(* This function block implements IEC60870-5-101 slave services *)
FUNCTION_BLOCK FB_IEC870_5_101SServices
VAR_IN_OUT
	stProcData 			: ST_IEC870_5_101SProcData;(* Process data send to or received from IEC 60870-5-101 slave device *)
	sysPara 			: ST_IEC870_5_101SSysPara;(* Local slave system parameters *)
	buffer				: ST_IEC870_5_101TBuffer;(* RX/TX buffer *)
	fbClock				: FB_LocalSystemTime;(* Internal clock: Local windows system time *)
	fbLog				: FB_IEC870_DebugLogFifo;(* Simple log buffer. We store/log here all our received slave data and other messages (for demonstration purpose only) *)
	bReset				: BOOL;(* Rising edge at this input resets service execution *)
END_VAR
VAR
	eState				: E_IEC870_5_101SState := e101SState_Init;(* Service/device execution state *)
	fbBuffer			: FB_IEC870_5_101TBufferCtrl; (* RX/TX buffer control function block *)
	txAsdu 				: ST_IEC870_5_101AOGen; (* Temp. asdu to send *)
	rxAsdu 				: ST_IEC870_5_101AOGen; (* Temp. received asdu *)
	fbSetLocalTime		: NT_SetLocalTime;

	fbCyclicTimer		: TON;(* Cyclic data timer *)
	fbCoroTimer			: TON;(* Local freeze/reset timer *)
	bGeninWait			: BOOL;(* TRUE => General interrogation in progress *)
	bCoroWait	 		: BOOL;(* TRUE => Counter interrogation in progress *)
	bEndOfInit			: BOOL;(* TRUE => End of initialization allready done *)

	st100 				: ST_IEC870_5_101SPendingState;(* Single point status flags *)
	st101 				: ST_IEC870_5_101SPendingState;(* Single point status flags *)
	st102 				: ST_IEC870_5_101SPendingState;(* Single point status flags *)
	st200 				: ST_IEC870_5_101SPendingState;(* Double point status flags *)
	st300 				: ST_IEC870_5_101SPendingState;(* Step position information status flags *)
	st400 				: ST_IEC870_5_101SPendingState;(* Bitstring status flags *)
	st500 				: ST_IEC870_5_101SPendingState;(* Measured value, normalized value status flags *)
	st600 				: ST_IEC870_5_101SPendingState;(* Measured value, scalled value status flags *)
	st700 				: ST_IEC870_5_101SPendingState;(* Measured value, short floating point number status flags *)
	st800 				: ST_IEC870_5_101SPendingState;(* Binary counter status flags *)
	st801 				: ST_IEC870_5_101SPendingState;(* Binary counter status flags *)
	st802 				: ST_IEC870_5_101SPendingState;(* Binary counter status flags *)
	
	stTxProcData		: ST_IEC870_5_101SProcData;
	
	(* Temporary variables *)
	tT56_new			: T_CP56Time2a;(* 56 bit time tag value *)
	tT56_old			: T_CP56Time2a;(* 56 bit time tag value *)
	tT24				: T_CP24Time2a;(* 24 bit time tag value *)
	tT56				: T_CP56Time2a;(* 56 bit time tag value *)
	stSiq				: ST_IEC870_5_101SIQ;(* Single point information + quality descriptor *)
	stDiq				: ST_IEC870_5_101DIQ;(* Double point information + quality descriptor *)
	stQds				: ST_IEC870_5_101QDS;(* Measured value quality descriptor *)
	stQcr				: ST_IEC870_5_101QCR;(* Binary counter quality descriptor *)

	nCoi				: BYTE;(* Cause of initialization *)
	eCoi				: E_IEC870_5_101COI := eIEC870_COI_LOCAL_POWER_ON;(* Cause of initialization as enumerated type *)
	
	nQoi				: BYTE;(* Qualifier of interrogation command *)	
	eQoi				: E_IEC870_5_101QOI;(* Qualifier of interrogation command as enumerated type *)
	
	nQcc				: BYTE;(* Qualifier of counter interrogation command *)
	eFrz				: E_IEC870_5_101FRZ;(* Counter interrogation freeze/reset qualifier *)
	eRqt				: E_IEC870_5_101RQT;(* Counter interrogation request qualifier *)

	nVti				: BYTE;(* Value with transient state indication *)
	nBsi				: DWORD;(* Bitstring information *)
	nNva				: WORD;(* Normalized value *)
	nSva				: INT;(* Scalled value *)
	fR32				: REAL;(* Short floating point value *)
	nBcr				: DINT;(* Binary counter reading *)
	
	nSco				: BYTE;(* Single command state + qualifier *)
	eScs				: E_IEC870_5_101SCS;(* Single command state *)
	
	nDco				: BYTE;(* Double command state + qualifier *)
	eDcs				: E_IEC870_5_101DCS;(* Double command state *)
	
	nRco				: BYTE;(* Regulating step command + qualifier *)
	eRcs				: E_IEC870_5_101RCS;(* Regulating step command *)
	
	eQu					: E_IEC870_5_101QU;(* Regulating step command qualifier *)
	nQos				: BYTE;(* Qualifier of setpoint command + select/execute flag *)
	eQl					: E_IEC870_5_101QL;(* Qualifier of setpoint command *)
	nFbp				: WORD := 16#55AA;(* Test command frame bit pattern activation data *)
	bSE					: BOOL;(* Select/execute flag (TRUE => Select, FALSE => Execute) *)
END_VAR

(* Please don't use the SIZEOF operator with CP56Time2a or CP24Time2a data type.
Because of the data alignment SIZEOF( tT56 ) or SIZEOF( tT24 ) leads to incorrect size. *)

IF bReset THEN(* Reset service execution *)
	bReset 	:= FALSE;
	MEMSET( ADR( st100 ), 0, SIZEOF( st100 ) );
	MEMSET( ADR( st101 ), 0, SIZEOF( st101 ) );
	MEMSET( ADR( st102 ), 0, SIZEOF( st102 ) );
	MEMSET( ADR( st200 ), 0, SIZEOF( st200 ) );
	MEMSET( ADR( st300 ), 0, SIZEOF( st300 ) );
	MEMSET( ADR( st400 ), 0, SIZEOF( st400 ) );
	MEMSET( ADR( st500 ), 0, SIZEOF( st500 ) );
	MEMSET( ADR( st600 ), 0, SIZEOF( st600 ) );
	MEMSET( ADR( st700 ), 0, SIZEOF( st700 ) );
	MEMSET( ADR( st800 ), 0, SIZEOF( st800 ) );
	MEMSET( ADR( st801 ), 0, SIZEOF( st801 ) );
	MEMSET( ADR( st802 ), 0, SIZEOF( st802 ) );
	fbCyclicTimer( IN := FALSE );(* Reset timer *)
	fbCoroTimer( IN := FALSE );(* Reset timer *)
	bGeninWait := FALSE;(* Reset flag *)
	bCoroWait := FALSE;(* Reset flag *)
	bEndOfInit := FALSE;(* Reset flag *)
	eState := e101SState_Init;
END_IF

(*-----------------------------------------------------------------------------------------*)
(* Simple implementation of cyclic data transfer *)
fbCyclicTimer( IN := sysPara.bCyclic, PT := sysPara.tCyclic );
IF fbCyclicTimer.Q THEN
	fbCyclicTimer( IN := FALSE ); 
	fbCyclicTimer( IN := sysPara.bCyclic );
	(* Set flags to force monitoring data to send cyclic data *)
	st100.bCyclic := TRUE;
	st101.bCyclic := TRUE;
	st102.bCyclic := TRUE;
	st200.bCyclic := TRUE;
	st300.bCyclic := TRUE;
	st400.bCyclic := TRUE;
	st500.bCyclic := TRUE;
	st600.bCyclic := TRUE;
	st700.bCyclic := TRUE;
END_IF
	
(*-----------------------------------------------------------------------------------------*)
(* Simple implementation of local counter freeze/reset functionality *)
IF ( sysPara.eCoroMode = eIEC870_CoroMode_A ) OR ( sysPara.eCoroMode = eIEC870_CoroMode_B ) THEN
	fbCoroTimer( IN := sysPara.bCoro, PT := sysPara.tCoro );
	IF fbCoroTimer.Q THEN
		fbCoroTimer( IN := FALSE ); 
		fbCoroTimer( IN := sysPara.bCoro );
		
		(* Freeze value *)
		stTxProcData.nBcr800 	:= stProcData.nBcr800;
		stTxProcData.nBcr801 	:= stProcData.nBcr801;
		stTxProcData.nBcr802 	:= stProcData.nBcr802;
		
		IF sysPara.bCoroReset THEN(* Reset value *)
			stProcData.nBcr800 		:= 0;
			stProcData.nBcr801 		:= 0;
			stProcData.nBcr802 		:= 0;
		END_IF
		
		IF sysPara.eCoroMode = eIEC870_CoroMode_A THEN(* Force spontaneous data transfer *)
			st800.bSpont := TRUE;
			st801.bSpont := TRUE;
			st802.bSpont := TRUE;
		END_IF
	
	END_IF
END_IF


(*-----------------------------------------------------------------------------------------*)
(* End of initialization *)
IF NOT bEndOfInit THEN
	(* Create asdu *)	
	txAsdu.ident.eType 		:= M_EI_NA_1;(* End of initialization *)
	txAsdu.ident.bSQ 		:= FALSE;
	txAsdu.ident.nObj 		:= 1;
	txAsdu.ident.eCOT 		:= eIEC870_COT_INIT;(* Set cause of transfer to initialization *)
	txAsdu.ident.nORG 		:= sysPara.nOrg;(* Set originator address *)
	txAsdu.ident.bPN 		:= FALSE;
	txAsdu.ident.bT 		:= FALSE;
	txAsdu.ident.eClass 	:= eIEC870_Class_1;(* Put to the high priority tx buffer *)
	txAsdu.ident.asduAddr 	:= sysPara.asduAddr;(* Set common asdu address *)
	txAsdu.info.objAddr		:= 0;(* Set information object address *)
	
	nCoi					:= INT_TO_BYTE( eCoi );
	nCoi.7 					:= FALSE;
	F_iecResetStream( 0, txAsdu.info.stream );(* Clear previous data (this sets the stream length = 0 *)
	F_iecCopyBufferToStream( ADR( nCoi ), SIZEOF( nCoi ), txAsdu.info.stream );(* Put COI to stream *)
	fbBuffer.TxAddObj( putObj := txAsdu, buffer := buffer );(* Put asdu to the TX fifo *)
	IF fbBuffer.bOk THEN(* Success *)
		fbLog.A_LogHint( sPut := CONCAT( '<=', IEC101ASDU_TO_STRING( txAsdu ) ) );(* Log data (for demonstration purpose only) *)
		bEndOfInit := TRUE;(* Set flag *)
	ELSE(* Report send buffer overflow warning *)
		fbLog.A_LogWarning( sPut := '::TX buffer overflow (end of initialization)!' );(* Log warning *)
	END_IF
END_IF

(*-----------------------------------------------------------------------------------------*)
(* Single-point, IOA := 100 *)
IF ( PBYTE_TO_BYTE( ADR( stProcData.stSiq100 ) ) <> PBYTE_TO_BYTE( ADR( stTxProcData.stSiq100 ) ) ) 
THEN(* Single-point information or quality flags changed *)
	st100.bSpont := TRUE;(* Force spontaneous data transfer *)
END_IF
IF st100.bSpont OR st100.bCyclic OR st100.bGenin THEN
	(* Create asdu *)
	txAsdu.ident.eType 		:= M_SP_NA_1;(* Single-point information *)
	txAsdu.ident.bSQ 		:= FALSE;
	txAsdu.ident.nObj 		:= 1;
	IF st100.bSpont THEN
		txAsdu.ident.eCOT 	:= eIEC870_COT_SPONTAN;(* Set cause of transfer to spontaneous *)
	ELSIF st100.bGenin THEN
		txAsdu.ident.eCOT 	:= QOI_TO_COT( eQoi );(* General interrogation data *)
	ELSIF st100.bCyclic THEN
		txAsdu.ident.eCOT 	:= eIEC870_COT_CYCLIC;(* Cyclic data *)
	END_IF
	txAsdu.ident.nORG 		:= sysPara.nOrg;(* Set originator address *)
	txAsdu.ident.bPN 		:= FALSE;
	txAsdu.ident.bT 		:= FALSE;
	txAsdu.ident.eClass 	:= SEL( st100.bCyclic, eIEC870_Class_1, eIEC870_Class_2 );(* Put cyclic data to the low priority and others to high priority tx buffer *)
	txAsdu.ident.asduAddr 	:= sysPara.asduAddr;(* Set common asdu address *)
	txAsdu.info.objAddr		:= 100;(* Set information object address *)
	
	stSiq					:= stProcData.stSiq100;
	F_iecResetStream( 0, txAsdu.info.stream );(* Clear previous data (this sets the stream length = 0 *)
	F_iecCopyBufferToStream( ADR( stSiq ), SIZEOF( stSiq ), txAsdu.info.stream );(* Put SIQ to stream *)
	fbBuffer.TxAddObj( putObj := txAsdu, buffer := buffer );(* Put asdu to the TX fifo *)
	IF fbBuffer.bOk THEN(* Success *)
		fbLog.A_LogHint( sPut := CONCAT( '<=', IEC101ASDU_TO_STRING( txAsdu ) ) );(* Log data (for demonstration purpose only) *)
		stTxProcData.stSiq100 := stSiq;
		IF st100.bSpont THEN
			st100.bSpont 	:= FALSE;
		ELSIF st100.bGenin THEN
			st100.bGenin 	:= FALSE;
		ELSIF st100.bCyclic THEN
			st100.bCyclic 	:= FALSE;
		END_IF
	ELSE(* Report send buffer overflow warning *)
		fbLog.A_LogWarning( sPut := '::TX buffer overflow (single-point information, IOA := 100)!' );(* Log warning *)
	END_IF
END_IF

(*-----------------------------------------------------------------------------------------*)
(* Single-point, IOA := 101 *)
IF ( PBYTE_TO_BYTE( ADR( stProcData.stSiq101 ) ) <> PBYTE_TO_BYTE( ADR( stTxProcData.stSiq101 ) ) ) 
THEN(* Single-point information or quality flags changed *)
	st101.bSpont := TRUE;(* Force spontaneous data transfer *)
END_IF
IF st101.bSpont OR st101.bCyclic OR st101.bGenin THEN
	(* Create asdu *)
	IF st101.bGenin THEN
		txAsdu.ident.eType 	:= M_SP_NA_1;(* Single-point information without time tag *)
	ELSE
		txAsdu.ident.eType 	:= M_SP_TA_1;(* Single-point information with 24 bit time tag *)
	END_IF
	txAsdu.ident.bSQ 		:= FALSE;
	txAsdu.ident.nObj 		:= 1;
	IF st101.bSpont THEN
		txAsdu.ident.eCOT 	:= eIEC870_COT_SPONTAN;(* Set cause of transfer to spontaneous *)
	ELSIF st101.bGenin THEN
		txAsdu.ident.eCOT 	:= QOI_TO_COT( eQoi );(* General interrogation data *)
	ELSIF st101.bCyclic THEN
		txAsdu.ident.eCOT 	:= eIEC870_COT_CYCLIC;(* Cyclic data *)
	END_IF
	txAsdu.ident.nORG 		:= sysPara.nOrg;(* Set originator address *)
	txAsdu.ident.bPN 		:= FALSE;
	txAsdu.ident.bT 		:= FALSE;
	txAsdu.ident.eClass 	:= SEL( st101.bCyclic, eIEC870_Class_1, eIEC870_Class_2 );(* Put cyclic data to the low priority and others to high priority tx buffer *)
	txAsdu.ident.asduAddr 	:= sysPara.asduAddr;(* Set common asdu address *)
	txAsdu.info.objAddr		:= 101;(* Set information object address *)
	
	stSiq					:= stProcData.stSiq101;
	tT24					:= CP56Time2a_TO_CP24Time2a( SYSTEMTIME_TO_CP56Time2a( fbClock.systemTime, fbClock.TzID = eTimeZoneID_Daylight ) );(* Send actual time stamp *)
	
	F_iecResetStream( 0, txAsdu.info.stream );(* Clear previous data (this sets the stream length = 0 *)
	F_iecCopyBufferToStream( ADR( stSiq ), SIZEOF( stSiq ), txAsdu.info.stream );(* Put SIQ to stream *)
	IF NOT st101.bGenin THEN
		F_iecCopyBufferToStream( ADR( tT24 ), 3(* SIZEOF( tT24 ) - 1 *), txAsdu.info.stream );(* Put time tag to stream *)
	END_IF
	fbBuffer.TxAddObj( putObj := txAsdu, buffer := buffer );(* Put asdu to the TX fifo *)
	IF fbBuffer.bOk THEN(* Success *)
		fbLog.A_LogHint( sPut := CONCAT( '<=', IEC101ASDU_TO_STRING( txAsdu ) ) );(* Log data (for demonstration purpose only) *)
		stTxProcData.stSiq101 := stSiq;
		IF st101.bSpont THEN
			st101.bSpont 	:= FALSE;
		ELSIF st101.bGenin THEN
			st101.bGenin 	:= FALSE;
		ELSIF st101.bCyclic THEN
			st101.bCyclic 	:= FALSE;
		END_IF
	ELSE(* Report send buffer overflow warning *)
		fbLog.A_LogWarning( sPut := '::TX buffer overflow (single-point information, IOA := 101)!' );(* Log warning *)
	END_IF
END_IF
(*-----------------------------------------------------------------------------------------*)
(* Single-point, IOA := 102 *)
IF ( PBYTE_TO_BYTE( ADR( stProcData.stSiq102 ) ) <> PBYTE_TO_BYTE( ADR( stTxProcData.stSiq102 ) ) ) 
THEN(* Single-point information or quality flags changed *)
	st102.bSpont := TRUE;(* Force spontaneous data transfer *)
END_IF
IF st102.bSpont OR st102.bCyclic OR st102.bGenin THEN
	(* Create asdu *)
	IF st102.bGenin THEN
		txAsdu.ident.eType 	:= M_SP_NA_1;(* Single-point information without time tag *)
	ELSE	
		txAsdu.ident.eType 	:= M_SP_TB_1;(* Single-point information with 56 bit time tag *)
	END_IF
	txAsdu.ident.bSQ 		:= FALSE;
	txAsdu.ident.nObj 		:= 1;
	IF st102.bSpont THEN
		txAsdu.ident.eCOT 	:= eIEC870_COT_SPONTAN;(* Set cause of transfer to spontaneous *)
	ELSIF st102.bGenin THEN
		txAsdu.ident.eCOT 	:= QOI_TO_COT( eQoi );(* General interrogation data *)
	ELSIF st102.bCyclic THEN
		txAsdu.ident.eCOT 	:= eIEC870_COT_CYCLIC;(* Cyclic data *)
	END_IF
	txAsdu.ident.nORG 		:= sysPara.nOrg;(* Set originator address *)
	txAsdu.ident.bPN 		:= FALSE;
	txAsdu.ident.bT 		:= FALSE;
	txAsdu.ident.eClass 	:= SEL( st102.bCyclic, eIEC870_Class_1, eIEC870_Class_2 );(* Put cyclic data to the low priority and others to high priority tx buffer *)
	txAsdu.ident.asduAddr 	:= sysPara.asduAddr;(* Set common asdu address *)
	txAsdu.info.objAddr		:= 102;(* Set information object address *)
	
	stSiq					:= stProcData.stSiq102;
	tT56					:= SYSTEMTIME_TO_CP56Time2a( fbClock.systemTime, fbClock.TzID = eTimeZoneID_Daylight );(* Send actual time stamp *)

	F_iecResetStream( 0, txAsdu.info.stream );(* Clear previous data (this sets the stream length = 0 *)
	F_iecCopyBufferToStream( ADR( stSiq ), SIZEOF( stSiq ), txAsdu.info.stream );(* Put SIQ to stream *)
	IF NOT st102.bGenin THEN
		F_iecCopyBufferToStream( ADR( tT56 ), 7(* SIZEOF( tT56 ) - 1 *), txAsdu.info.stream );(* Put time tag to stream *)
	END_IF
	fbBuffer.TxAddObj( putObj := txAsdu, buffer := buffer );(* Put asdu to the TX fifo *)
	IF fbBuffer.bOk THEN(* Success *)
		fbLog.A_LogHint( sPut := CONCAT( '<=', IEC101ASDU_TO_STRING( txAsdu ) ) );(* Log data (for demonstration purpose only) *)
		stTxProcData.stSiq102 := stSiq;
		IF st102.bSpont THEN
			st102.bSpont 	:= FALSE;
		ELSIF st102.bGenin THEN
			st102.bGenin 	:= FALSE;
		ELSIF st102.bCyclic THEN
			st102.bCyclic 	:= FALSE;
		END_IF
	ELSE(* Report send buffer overflow warning *)
		fbLog.A_LogWarning( sPut := '::TX buffer overflow (single-point information, IOA := 102)!' );(* Log warning *)
	END_IF
END_IF



(*-----------------------------------------------------------------------------------------*)
(* Double-point, IOA := 200 *)
IF ( PBYTE_TO_BYTE( ADR( stProcData.stDiq200 ) ) <> PBYTE_TO_BYTE( ADR( stTxProcData.stDiq200 ) ) ) 
THEN(* Double-point information or quality flags changed *)
	st200.bSpont := TRUE;(* Force spontaneous data transfer *)
END_IF
IF st200.bSpont OR st200.bCyclic OR st200.bGenin THEN
	(* Create asdu *)
	txAsdu.ident.eType 		:= M_DP_NA_1;(* Double-point information *)
	txAsdu.ident.bSQ 		:= FALSE;
	txAsdu.ident.nObj 		:= 1;
	IF st200.bSpont THEN
		txAsdu.ident.eCOT 	:= eIEC870_COT_SPONTAN;(* Set cause of transfer to spontaneous *)
	ELSIF st200.bGenin THEN
		txAsdu.ident.eCOT 	:= QOI_TO_COT( eQoi );(* General interrogation data *)
	ELSIF st200.bCyclic THEN
		txAsdu.ident.eCOT 	:= eIEC870_COT_CYCLIC;(* Cyclic data *)
	END_IF
	txAsdu.ident.nORG 		:= sysPara.nOrg;(* Set originator address *)
	txAsdu.ident.bPN 		:= FALSE;
	txAsdu.ident.bT 		:= FALSE;
	txAsdu.ident.eClass 	:= SEL( st200.bCyclic, eIEC870_Class_1, eIEC870_Class_2 );(* Put cyclic data to the low priority and others to high priority tx buffer *)
	txAsdu.ident.asduAddr 	:= sysPara.asduAddr;(* Set common asdu address *)
	txAsdu.info.objAddr		:= 200;(* Set information object address *)
	
	stDiq 					:= stProcData.stDiq200;
	F_iecResetStream( 0, txAsdu.info.stream );(* Clear previous data (this sets the stream length = 0 *)
	F_iecCopyBufferToStream( ADR( stDiq ), SIZEOF( stDiq ), txAsdu.info.stream );(* Put DIQ to stream *)
	fbBuffer.TxAddObj( putObj := txAsdu, buffer := buffer );(* Put asdu to the TX fifo *)
	IF fbBuffer.bOk THEN(* Success *)
		fbLog.A_LogHint( sPut := CONCAT( '<=', IEC101ASDU_TO_STRING( txAsdu ) ) );(* Log data (for demonstration purpose only) *)
		stTxProcData.stDiq200 := stDiq;
		IF st200.bSpont THEN
			st200.bSpont 	:= FALSE;
		ELSIF st200.bGenin THEN
			st200.bGenin 	:= FALSE;
		ELSIF st200.bCyclic THEN
			st200.bCyclic 	:= FALSE;
		END_IF
	ELSE(* Report send buffer overflow warning *)
		fbLog.A_LogWarning( sPut := '::TX buffer overflow (double-point information)!' );(* Log warning *)
	END_IF
END_IF

(*-----------------------------------------------------------------------------------------*)
(* Step position *)
IF ( stProcData.nVti300 <> stTxProcData.nVti300 ) 
OR ( PBYTE_TO_BYTE( ADR( stProcData.stQds300 ) ) <> PBYTE_TO_BYTE( ADR( stTxProcData.stQds300 ) ) ) 
THEN(* Value with transient state or quality flags changed *)
	st300.bSpont := TRUE;(* Force spontaneous data transfer *)
END_IF
IF st300.bSpont OR st300.bCyclic OR st300.bGenin THEN
	(* Create asdu *)
	txAsdu.ident.eType 		:= M_ST_NA_1;(* Step position information *)
	txAsdu.ident.bSQ 		:= FALSE;
	txAsdu.ident.nObj 		:= 1;
	IF st300.bSpont THEN
		txAsdu.ident.eCOT 	:= eIEC870_COT_SPONTAN;(* Set cause of transfer to spontaneous *)
	ELSIF st300.bGenin THEN
		txAsdu.ident.eCOT 	:= QOI_TO_COT( eQoi );(* General interrogation data *)
	ELSIF st300.bCyclic THEN
		txAsdu.ident.eCOT 	:= eIEC870_COT_CYCLIC;(* Cyclic data *)
	END_IF
	txAsdu.ident.nORG 		:= sysPara.nOrg;(* Set originator address *)
	txAsdu.ident.bPN 		:= FALSE;
	txAsdu.ident.bT 		:= FALSE;
	txAsdu.ident.eClass 	:= SEL( st300.bCyclic, eIEC870_Class_1, eIEC870_Class_2 );(* Put cyclic data to the low priority and others to high priority tx buffer *)
	txAsdu.ident.asduAddr 	:= sysPara.asduAddr;(* Set common asdu address *)
	txAsdu.info.objAddr		:= 300;(* Set information object address *)
	
	nVti 					:= stProcData.nVti300;
	stQds 					:= stProcData.stQds300;
	F_iecResetStream( 0, txAsdu.info.stream );(* Clear previous data (this sets the stream length = 0 *)
	F_iecCopyBufferToStream( ADR( nVti ), SIZEOF( nVti ), txAsdu.info.stream );(* Put VTI to stream *)
	F_iecCopyBufferToStream( ADR( stQds ), SIZEOF( stQds ), txAsdu.info.stream );(* Put QDS to stream *)
	fbBuffer.TxAddObj( putObj := txAsdu, buffer := buffer );(* Put asdu to the TX fifo *)
	IF fbBuffer.bOk THEN(* Success *)
		fbLog.A_LogHint( sPut := CONCAT( '<=', IEC101ASDU_TO_STRING( txAsdu ) ) );(* Log data (for demonstration purpose only) *)
		stTxProcData.nVti300 	:= nVti;
		stTxProcData.stQds300 	:= stQds;
		IF st300.bSpont THEN
			st300.bSpont 	:= FALSE;
		ELSIF st300.bGenin THEN
			st300.bGenin 	:= FALSE;
		ELSIF st300.bCyclic THEN
			st300.bCyclic 	:= FALSE;
		END_IF
	ELSE(* Report send buffer overflow warning *)
		fbLog.A_LogWarning( sPut := '::TX buffer overflow (step position information)!' );(* Log warning *)
	END_IF
END_IF

(*-----------------------------------------------------------------------------------------*)
(* Bitstring *)
IF ( stProcData.nBsi400 <> stTxProcData.nBsi400 )
OR ( PBYTE_TO_BYTE( ADR( stProcData.stQds400 ) ) <> PBYTE_TO_BYTE( ADR( stTxProcData.stQds400 ) ) ) 
THEN(* Bistring value or quality flags changed *)
	st400.bSpont := TRUE;(* Force spontaneous data transfer *)
END_IF
IF st400.bSpont OR st400.bCyclic OR st400.bGenin THEN
	(* Create asdu *)
	txAsdu.ident.eType 		:= M_BO_NA_1;(* Bitstring of 32 bit *)
	txAsdu.ident.bSQ 		:= FALSE;
	txAsdu.ident.nObj 		:= 1;
	IF st400.bSpont THEN
		txAsdu.ident.eCOT 	:= eIEC870_COT_SPONTAN;(* Set cause of transfer to spontaneous *)
	ELSIF st400.bGenin THEN
		txAsdu.ident.eCOT 	:= QOI_TO_COT( eQoi );(* General interrogation data *)
	ELSIF st400.bCyclic THEN
		txAsdu.ident.eCOT 	:= eIEC870_COT_CYCLIC;(* Cyclic data *)
	END_IF
	txAsdu.ident.nORG 		:= sysPara.nOrg;(* Set originator address *)
	txAsdu.ident.bPN 		:= FALSE;
	txAsdu.ident.bT 		:= FALSE;
	txAsdu.ident.eClass 	:= SEL( st400.bCyclic, eIEC870_Class_1, eIEC870_Class_2 );(* Put cyclic data to the low priority and others to high priority tx buffer *)
	txAsdu.ident.asduAddr 	:= sysPara.asduAddr;(* Set common asdu address *)
	txAsdu.info.objAddr		:= 400;(* Set information object address *)
	
	nBsi 					:= stProcData.nBsi400;
	stQds					:= stProcData.stQds400;
	F_iecResetStream( 0, txAsdu.info.stream );(* Clear previous data (this sets the stream length = 0 *)
	F_iecCopyBufferToStream( ADR( nBsi ), SIZEOF( nBsi ), txAsdu.info.stream );(* Put BSI to stream *)
	F_iecCopyBufferToStream( ADR( stQds ), SIZEOF( stQds ), txAsdu.info.stream );(* Put QDS to stream *)
	fbBuffer.TxAddObj( putObj := txAsdu, buffer := buffer );(* Put asdu to the TX fifo *)
	IF fbBuffer.bOk THEN(* Success *)
		fbLog.A_LogHint( sPut := CONCAT( '<=', IEC101ASDU_TO_STRING( txAsdu ) ) );(* Log data (for demonstration purpose only) *)
		stTxProcData.nBsi400 	:= nBsi;
		stTxProcData.stQds400 	:= stQds;
		IF st400.bSpont THEN
			st400.bSpont 	:= FALSE;
		ELSIF st400.bGenin THEN
			st400.bGenin 	:= FALSE;
		ELSIF st400.bCyclic THEN
			st400.bCyclic 	:= FALSE;
		END_IF
	ELSE(* Report send buffer overflow warning *)
		fbLog.A_LogWarning( sPut := '::TX buffer overflow (bitstring information)!' );(* Log warning *)
	END_IF
END_IF

(*-----------------------------------------------------------------------------------------*)
(* Measured value, normalized value *)
IF ( stProcData.nNva500 <> stTxProcData.nNva500 )
OR ( PBYTE_TO_BYTE( ADR( stProcData.stQds500 ) ) <> PBYTE_TO_BYTE( ADR( stTxProcData.stQds500 ) ) ) 
THEN(* Measured value or quality flags changed *)
	st500.bSpont := TRUE;(* Force spontaneous data transfer *)
END_IF
IF st500.bSpont OR st500.bCyclic OR st500.bGenin THEN
	(* Create asdu *)
	txAsdu.ident.eType 		:= M_ME_NA_1;(* Normalized value *)
	txAsdu.ident.bSQ 		:= FALSE;
	txAsdu.ident.nObj 		:= 1;
	IF st500.bSpont THEN
		txAsdu.ident.eCOT 	:= eIEC870_COT_SPONTAN;(* Set cause of transfer to spontaneous *)
	ELSIF st500.bGenin THEN
		txAsdu.ident.eCOT 	:= QOI_TO_COT( eQoi );(* General interrogation data *)
	ELSIF st500.bCyclic THEN
		txAsdu.ident.eCOT 	:= eIEC870_COT_CYCLIC;(* Cyclic data *)
	END_IF
	txAsdu.ident.nORG 		:= sysPara.nOrg;(* Set originator address *)
	txAsdu.ident.bPN 		:= FALSE;
	txAsdu.ident.bT 		:= FALSE;
	txAsdu.ident.eClass 	:= SEL( st500.bCyclic, eIEC870_Class_1, eIEC870_Class_2 );(* Put cyclic data to the low priority and others to high priority tx buffer *)
	txAsdu.ident.asduAddr 	:= sysPara.asduAddr;(* Set common asdu address *)
	txAsdu.info.objAddr		:= 500;(* Set information object address *)
	
	nNva 					:= stProcData.nNva500;
	stQds					:= stProcData.stQds500;
	F_iecResetStream( 0, txAsdu.info.stream );(* Clear previous data (this sets the stream length = 0 *)
	F_iecCopyBufferToStream( ADR( nNva ), SIZEOF( nNva ), txAsdu.info.stream );(* Put NVA to stream *)
	F_iecCopyBufferToStream( ADR( stQds ), SIZEOF( stQds ), txAsdu.info.stream );(* Put QDS to stream *)
	fbBuffer.TxAddObj( putObj := txAsdu, buffer := buffer );(* Put asdu to the TX fifo *)
	IF fbBuffer.bOk THEN(* Success *)
		fbLog.A_LogHint( sPut := CONCAT( '<=', IEC101ASDU_TO_STRING( txAsdu ) ) );(* Log data (for demonstration purpose only) *)
		stTxProcData.nNva500 	:= nNva;
		stTxProcData.stQds500 	:= stQds;
		IF st500.bSpont THEN
			st500.bSpont 	:= FALSE;
		ELSIF st500.bGenin THEN
			st500.bGenin 	:= FALSE;
		ELSIF st500.bCyclic THEN
			st500.bCyclic 	:= FALSE;
		END_IF
	ELSE(* Report send buffer overflow warning *)
		fbLog.A_LogWarning( sPut := '::TX buffer overflow (normalized value)!' );(* Log warning *)
	END_IF
END_IF

(*-----------------------------------------------------------------------------------------*)
(* Measured value, scalled value *)
IF ( stProcData.nSva600 <> stTxProcData.nSva600 )
OR ( PBYTE_TO_BYTE( ADR( stProcData.stQds600 ) ) <> PBYTE_TO_BYTE( ADR( stTxProcData.stQds600 ) ) ) 
THEN(* Measured value or quality flags changed *)
	st600.bSpont := TRUE;(* Force spontaneous data transfer *)
END_IF
IF st600.bSpont OR st600.bCyclic OR st600.bGenin THEN
	(* Create asdu *)
	txAsdu.ident.eType 		:= M_ME_NB_1;(* Scalled value *)
	txAsdu.ident.bSQ 		:= FALSE;
	txAsdu.ident.nObj 		:= 1;
	IF st600.bSpont THEN
		txAsdu.ident.eCOT 	:= eIEC870_COT_SPONTAN;(* Set cause of transfer to spontaneous *)
	ELSIF st600.bGenin THEN
		txAsdu.ident.eCOT 	:= QOI_TO_COT( eQoi );(* General interrogation data *)
	ELSIF st600.bCyclic THEN
		txAsdu.ident.eCOT 	:= eIEC870_COT_CYCLIC;(* Cyclic data *)
	END_IF
	txAsdu.ident.nORG 		:= sysPara.nOrg;(* Set originator address *)
	txAsdu.ident.bPN 		:= FALSE;
	txAsdu.ident.bT 		:= FALSE;
	txAsdu.ident.eClass 	:= SEL( st600.bCyclic, eIEC870_Class_1, eIEC870_Class_2 );(* Put cyclic data to the low priority and others to high priority tx buffer *)
	txAsdu.ident.asduAddr 	:= sysPara.asduAddr;(* Set common asdu address *)
	txAsdu.info.objAddr		:= 600;(* Set information object address *)
	
	nSva 					:= stProcData.nSva600;
	stQds					:= stProcData.stQds600;
	F_iecResetStream( 0, txAsdu.info.stream );(* Clear previous data (this sets the stream length = 0 *)
	F_iecCopyBufferToStream( ADR( nSva ), SIZEOF( nSva ), txAsdu.info.stream );(* Put SVA to stream *)
	F_iecCopyBufferToStream( ADR( stQds ), SIZEOF( stQds ), txAsdu.info.stream );(* Put QDS to stream *)
	fbBuffer.TxAddObj( putObj := txAsdu, buffer := buffer );(* Put asdu to the TX fifo *)
	IF fbBuffer.bOk THEN(* Success *)
		fbLog.A_LogHint( sPut := CONCAT( '<=', IEC101ASDU_TO_STRING( txAsdu ) ) );(* Log data (for demonstration purpose only) *)
		stTxProcData.nSva600 	:= nSva;
		stTxProcData.stQds600 	:= stQds;
		IF st600.bSpont THEN
			st600.bSpont 	:= FALSE;
		ELSIF st600.bGenin THEN
			st600.bGenin 	:= FALSE;
		ELSIF st600.bCyclic THEN
			st600.bCyclic 	:= FALSE;
		END_IF
	ELSE(* Report send buffer overflow warning *)
		fbLog.A_LogWarning( sPut := '::TX buffer overflow (scalled value)!' );(* Log warning *)
	END_IF
END_IF

(*-----------------------------------------------------------------------------------------*)
(* Measured value, short floating point value *)
IF ( stProcData.fSingle700 <> stTxProcData.fSingle700 )
OR ( PBYTE_TO_BYTE( ADR( stProcData.stQds700 ) ) <> PBYTE_TO_BYTE( ADR( stTxProcData.stQds700 ) ) ) 
THEN(* Measured value or quality flags changed *)
	st700.bSpont := TRUE;(* Force spontaneous data transfer *)
END_IF
IF st700.bSpont OR st700.bCyclic OR st700.bGenin THEN
	(* Create asdu *)
	txAsdu.ident.eType 		:= M_ME_NC_1;(* Short floating point value *)
	txAsdu.ident.bSQ 		:= FALSE;
	txAsdu.ident.nObj 		:= 1;
	IF st700.bSpont THEN
		txAsdu.ident.eCOT 	:= eIEC870_COT_SPONTAN;(* Set cause of transfer to spontaneous *)
	ELSIF st700.bGenin THEN
		txAsdu.ident.eCOT 	:= QOI_TO_COT( eQoi );(* General interrogation data *)
	ELSIF st700.bCyclic THEN
		txAsdu.ident.eCOT 	:= eIEC870_COT_CYCLIC;(* Cyclic data *)
	END_IF
	txAsdu.ident.nORG 		:= sysPara.nOrg;(* Set originator address *)
	txAsdu.ident.bPN 		:= FALSE;
	txAsdu.ident.bT 		:= FALSE;
	txAsdu.ident.eClass 	:= SEL( st700.bCyclic, eIEC870_Class_1, eIEC870_Class_2 );(* Put cyclic data to the low priority and others to high priority tx buffer *)
	txAsdu.ident.asduAddr 	:= sysPara.asduAddr;(* Set common asdu address *)
	txAsdu.info.objAddr		:= 700;(* Set information object address *)
	
	fR32 					:= stProcData.fSingle700;
	stQds					:= stProcData.stQds700;
	F_iecResetStream( 0, txAsdu.info.stream );(* Clear previous data (this sets the stream length = 0 *)
	F_iecCopyBufferToStream( ADR( fR32 ), SIZEOF( fR32 ), txAsdu.info.stream );(* Put R32 to stream *)
	F_iecCopyBufferToStream( ADR( stQds ), SIZEOF( stQds ), txAsdu.info.stream );(* Put QDS to stream *)
	fbBuffer.TxAddObj( putObj := txAsdu, buffer := buffer );(* Put asdu to the TX fifo *)
	IF fbBuffer.bOk THEN(* Success *)
		fbLog.A_LogHint( sPut := CONCAT( '<=', IEC101ASDU_TO_STRING( txAsdu ) ) );(* Log data (for demonstration purpose only) *)
		stTxProcData.fSingle700 := fR32;
		stTxProcData.stQds700 	:= stQds;
		IF st700.bSpont THEN
			st700.bSpont 	:= FALSE;
		ELSIF st700.bGenin THEN
			st700.bGenin 	:= FALSE;
		ELSIF st700.bCyclic THEN
			st700.bCyclic 	:= FALSE;
		END_IF
	ELSE(* Report send buffer overflow warning *)
		fbLog.A_LogWarning( sPut := '::TX buffer overflow (short floating point value)!' );(* Log warning *)
	END_IF
END_IF



(*-----------------------------------------------------------------------------------------*)
(* Binary counter value, IOA := 800 *)
IF ( PBYTE_TO_BYTE( ADR( stProcData.stQcr800 ) ) <> PBYTE_TO_BYTE( ADR( stTxProcData.stQcr800 ) ) ) 
THEN(* Quality flags changed *)
	stTxProcData.stQcr800 := stProcData.stQcr800;(* Save new quality flags *)
	st800.bSpont := TRUE;(* Force spontaneous data transfer *)
END_IF
IF st800.bSpont OR st800.bCoro THEN
	(* Create asdu *)
	txAsdu.ident.eType 		:= M_IT_NA_1;(* Binary counter read without time tag! *)
	txAsdu.ident.bSQ 		:= FALSE;
	txAsdu.ident.nObj 		:= 1;
	IF st800.bSpont THEN
		txAsdu.ident.eCOT 	:= eIEC870_COT_SPONTAN;(* Set cause of transfer to spontaneous *)
	ELSIF st800.bCoro THEN
		txAsdu.ident.eCOT 	:= RQT_TO_COT( eRqt );(* Set cause of transfer to interrogated by counter interrogation*)
	END_IF
	txAsdu.ident.nORG 		:= sysPara.nOrg;(* Set originator address *)
	txAsdu.ident.bPN 		:= FALSE;
	txAsdu.ident.bT 		:= FALSE;
	txAsdu.ident.eClass 	:= eIEC870_Class_1;(* Put to the high priority tx buffer *)
	txAsdu.ident.asduAddr 	:= sysPara.asduAddr;(* Set common asdu address *)
	txAsdu.info.objAddr		:= 800;(* Set information object address *)

	nBcr 					:= stTxProcData.nBcr800;(* Send freeze/reset value *)
	stQcr					:= stTxProcData.stQcr800;(* Send latest quality flags *)
	
	F_iecResetStream( 0, txAsdu.info.stream );(* Clear previous data (this sets the stream length = 0 *)
	F_iecCopyBufferToStream( ADR( nBcr ), SIZEOF( nBcr ), txAsdu.info.stream );(* Put BCR to stream *)
	F_iecCopyBufferToStream( ADR( stQcr ), SIZEOF( stQcr ), txAsdu.info.stream );(* Put quality to stream *)
	fbBuffer.TxAddObj( putObj := txAsdu, buffer := buffer );(* put asdu to the TX fifo *)
	IF fbBuffer.bOk THEN
		fbLog.A_LogHint( sPut := CONCAT( '<=', IEC101ASDU_TO_STRING(txAsdu) ) );
		IF st800.bSpont THEN
			st800.bSpont 	:= FALSE;
		ELSIF st800.bCoro THEN
			st800.bCoro 	:= FALSE;
		END_IF 
	ELSE(* Report send buffer overflow warning *)
		fbLog.A_LogWarning( sPut := '::TX buffer overflow (counter data)!' );
	END_IF
END_IF

(*-----------------------------------------------------------------------------------------*)
(* Binary counter value, IOA := 801 *)
IF ( PBYTE_TO_BYTE( ADR( stProcData.stQcr801 ) ) <> PBYTE_TO_BYTE( ADR( stTxProcData.stQcr801 ) ) ) 
THEN(* Quality flags changed *)
	stTxProcData.stQcr801 := stProcData.stQcr801;(* Save new quality flags *)
	st801.bSpont := TRUE;(* Force spontaneous data transfer *)
END_IF
IF st801.bSpont OR st801.bCoro THEN
	(* Create asdu *)
	txAsdu.ident.eType 		:= M_IT_TA_1;(* Binary counter read without time tag! *)
	txAsdu.ident.bSQ 		:= FALSE;
	txAsdu.ident.nObj 		:= 1;
	IF st801.bSpont THEN
		txAsdu.ident.eCOT 	:= eIEC870_COT_SPONTAN;(* Set cause of transfer to spontaneous *)
	ELSIF st801.bCoro THEN
		txAsdu.ident.eCOT 	:= RQT_TO_COT( eRqt );(* Set cause of transfer to interrogated by counter interrogation*)
	END_IF
	txAsdu.ident.nORG 		:= sysPara.nOrg;(* Set originator address *)
	txAsdu.ident.bPN 		:= FALSE;
	txAsdu.ident.bT 		:= FALSE;
	txAsdu.ident.eClass 	:= eIEC870_Class_1;(* Put to the high priority tx buffer *)
	txAsdu.ident.asduAddr 	:= sysPara.asduAddr;(* Set common asdu address *)
	txAsdu.info.objAddr		:= 801;(* Set information object address *)

	nBcr 					:= stTxProcData.nBcr801;(* Send freeze/reset value *)
	stQcr					:= stTxProcData.stQcr801;(* Send latest quality flags *)
	tT24					:= CP56Time2a_TO_CP24Time2a( SYSTEMTIME_TO_CP56Time2a( fbClock.systemTime, fbClock.TzID = eTimeZoneID_Daylight ) );(* Send actual time stamp *)
	
	F_iecResetStream( 0, txAsdu.info.stream );(* Clear previous data (this sets the stream length = 0 *)
	F_iecCopyBufferToStream( ADR( nBcr ), SIZEOF( nBcr ), txAsdu.info.stream );(* Put BCR to stream *)
	F_iecCopyBufferToStream( ADR( stQcr ), SIZEOF( stQcr ), txAsdu.info.stream );(* Put quality to stream *)
	F_iecCopyBufferToStream( ADR( tT24 ), 3(* SIZEOF( tT24 ) - 1 *), txAsdu.info.stream );(* Put quality to stream *)
	fbBuffer.TxAddObj( putObj := txAsdu, buffer := buffer );(* put asdu to the TX fifo *)
	IF fbBuffer.bOk THEN
		fbLog.A_LogHint( sPut := CONCAT( '<=', IEC101ASDU_TO_STRING(txAsdu) ) );
		IF st801.bSpont THEN
			st801.bSpont 	:= FALSE;
		ELSIF st801.bCoro THEN
			st801.bCoro 	:= FALSE;
		END_IF 
	ELSE(* Report send buffer overflow warning *)
		fbLog.A_LogWarning( sPut := '::TX buffer overflow (counter data)!' );
	END_IF
END_IF

(*-----------------------------------------------------------------------------------------*)
(* Binary counter value, IOA := 802 *)
IF ( PBYTE_TO_BYTE( ADR( stProcData.stQcr802 ) ) <> PBYTE_TO_BYTE( ADR( stTxProcData.stQcr802 ) ) ) 
THEN(* Quality flags changed *)
	stTxProcData.stQcr802 := stProcData.stQcr802;(* Save new quality flags *)
	st802.bSpont := TRUE;(* Force spontaneous data transfer *)
END_IF
IF st802.bSpont OR st802.bCoro THEN
	(* Create asdu *)
	txAsdu.ident.eType 		:= M_IT_TB_1;(* Binary counter read without time tag! *)
	txAsdu.ident.bSQ 		:= FALSE;
	txAsdu.ident.nObj 		:= 1;
	IF st802.bSpont THEN
		txAsdu.ident.eCOT 	:= eIEC870_COT_SPONTAN;(* Set cause of transfer to spontaneous *)
	ELSIF st802.bCoro THEN
		txAsdu.ident.eCOT 	:= RQT_TO_COT( eRqt );(* Set cause of transfer to interrogated by counter interrogation*)
	END_IF
	txAsdu.ident.nORG 		:= sysPara.nOrg;(* Set originator address *)
	txAsdu.ident.bPN 		:= FALSE;
	txAsdu.ident.bT 		:= FALSE;
	txAsdu.ident.eClass 	:= eIEC870_Class_1;(* Put to the high priority tx buffer *)
	txAsdu.ident.asduAddr 	:= sysPara.asduAddr;(* Set common asdu address *)
	txAsdu.info.objAddr		:= 802;(* Set information object address *)

	nBcr 					:= stTxProcData.nBcr802;(* Send freeze/reset value *)
	stQcr					:= stTxProcData.stQcr802;(* Send latest quality flags *)
	tT56					:= SYSTEMTIME_TO_CP56Time2a( fbClock.systemTime, fbClock.TzID = eTimeZoneID_Daylight );(* Send actual time stamp *)
	
	F_iecResetStream( 0, txAsdu.info.stream );(* Clear previous data (this sets the stream length = 0 *)
	F_iecCopyBufferToStream( ADR( nBcr ), SIZEOF( nBcr ), txAsdu.info.stream );(* Put BCR to stream *)
	F_iecCopyBufferToStream( ADR( stQcr ), SIZEOF( stQcr ), txAsdu.info.stream );(* Put quality to stream *)
	F_iecCopyBufferToStream( ADR( tT56 ), 7(* SIZEOF( tT56 ) - 1 *), txAsdu.info.stream );(* Put time tag to stream *)
	fbBuffer.TxAddObj( putObj := txAsdu, buffer := buffer );(* put asdu to the TX fifo *)
	IF fbBuffer.bOk THEN
		fbLog.A_LogHint( sPut := CONCAT( '<=', IEC101ASDU_TO_STRING(txAsdu) ) );
		IF st802.bSpont THEN
			st802.bSpont 	:= FALSE;
		ELSIF st802.bCoro THEN
			st802.bCoro 	:= FALSE;
		END_IF 
	ELSE(* Report send buffer overflow warning *)
		fbLog.A_LogWarning( sPut := '::TX buffer overflow (counter data)!' );
	END_IF
END_IF


(*-----------------------------------------------------------------------------------------*)
(* Perform the execution of received master commands *)
CASE eState OF
	e101SState_Init:(* Get next received (command) asdu *)
		fbBuffer.RxRemoveObj( getObj=>rxAsdu, buffer := buffer );(* Try to remove asdu from RX fifo *)
		IF fbBuffer.bOk THEN(* Success *)
			fbLog.A_LogHint( sPut := CONCAT( '=>', IEC101ASDU_TO_STRING( rxAsdu ) ) );(* Log data (for demonstration purpose only) *)
			CASE rxAsdu.ident.eType OF
				C_TS_NA_1:(* Test command *)
					eState := e101SState_TestAct;
				C_CS_NA_1:(* Clock synchronisation command *)
					eState := e101SState_ClockAct;
				C_IC_NA_1:(* General interrogation command *)
					eState := e101SState_GeninAct;
				C_CI_NA_1:(* Counter interrogation command*)
					eState := e101SState_CoroAct;
				C_SC_NA_1, C_SC_TA_1:(* Single command *)
					eState := e101SState_ScsCmdAct;
				C_DC_NA_1, C_DC_TA_1:(* Double command *)
					eState := e101SState_DcsCmdAct;
				C_RC_NA_1, C_RC_TA_1:(* Regulating step command *)
					eState := e101SState_RcsCmdAct;
				C_BO_NA_1, C_BO_TA_1:(* Bitstring command *)
					eState := e101SState_BsiCmdAct;
				C_SE_NA_1, C_SE_TA_1:(* Set-point command, normalized value *)
					eState := e101SState_NvaCmdAct;
				C_SE_NB_1, C_SE_TB_1:(* Set-point command, scalled value *)
					eState := e101SState_SvaCmdAct;
				C_SE_NC_1, C_SE_TC_1:(* Set-point command, short floating point number *)
					eState := e101SState_R32CmdAct;
				C_CD_NA_1:(* Delay acquisition command *)
					IF rxAsdu.ident.eCOT = eIEC870_COT_ACT THEN
						eState := e101SState_DelayAct;
					ELSIF rxAsdu.ident.eCOT = eIEC870_COT_SPONTAN THEN
						eState := e101SState_DelaySpt;
					END_IF
			ELSE(* Report invalid/not supported asdu type *)
				fbLog.A_LogWarning( sPut := '::Unusupported asdu type!' );
			END_CASE
		END_IF

	(*-----------------------------------------------------------------------------------------*)
	e101SState_TestAct:(* Test command activation *)
		F_iecCopyStreamToBuffer( ADR( nFbp ), SIZEOF( nFbp ), rxAsdu.info.stream );(* Copy FBP value to local variable *)
		eState := e101SState_TestCon;(* Send test command *)
	(*-----------------------------------------------------------------------------------------*)
	e101SState_TestCon:(* Test command activation confirmation *)
		txAsdu := rxAsdu;(* Create asdu *)
		txAsdu.ident.eCOT := eIEC870_COT_ACT_CON;(* Send activation confirmation *)
		fbBuffer.TxAddObj( putObj := txAsdu, buffer := buffer );(* Put asdu to the TX fifo *)
		IF fbBuffer.bOk THEN(* Success *)
			fbLog.A_LogHint( sPut := CONCAT( '<=', IEC101ASDU_TO_STRING(txAsdu) ) );(* Log data (for demonstration purpose only) *)
			eState := e101SState_Init;
		ELSE(* Report send buffer overflow warning *)
			fbLog.A_LogWarning( sPut := '::TX buffer overflow (test command activation confirmation)!' );
		END_IF
	(*-----------------------------------------------------------------------------------------*)
	e101SState_ClockAct:(* Clock synchronisation command activation *)
		F_iecCopyStreamToBuffer( ADR( tT56_new ), 7(* SIZEOF( tT56_new ) - 1 *), rxAsdu.info.stream );(* Get new time *)

		tT56_old := SYSTEMTIME_TO_CP56Time2a( fbClock.systemTime, fbClock.TzID = eTimeZoneID_Daylight );(* Get old time *)
		
		(* TODO: e.g. set your local (windows) system time *)
		fbSetLocalTime( START := FALSE );
		fbSetLocalTime( TIMESTR := CP56Time2a_TO_SYSTEMTIME( tT56_new, 20 ), START := TRUE );
		eState := e101SState_ClockSet;		
	(*-----------------------------------------------------------------------------------------*)
	e101SState_ClockSet:(* Wait until fbSetLocalTime() is not busy *)
		fbSetLocalTime( START := FALSE );
		IF NOT fbSetLocalTime.BUSY THEN
			IF fbSetLocalTime.ERR THEN(* Report error *)
				fbLog.A_LogError( sPut := '::NT_SetLocalTime() failed!' );
			END_IF
			eState := e101SState_ClockCon;		
		END_IF
	(*-----------------------------------------------------------------------------------------*)
	e101SState_ClockCon:(* Clock synchronisation command activation confirmation *)
		txAsdu := rxAsdu;(* Create asdu *)
		txAsdu.ident.eCOT := eIEC870_COT_ACT_CON;(* Send activation confirmation *)
		F_iecResetStream( 0, txAsdu.info.stream );(* Clear previous data (this sets the stream length = 0 *)
		F_iecCopyBufferToStream( ADR( tT56_old ), 7(* SIZEOF( tT56_old ) - 1 *), txAsdu.info.stream );(* Put old time to stream *)
		fbBuffer.TxAddObj( putObj := txAsdu, buffer := buffer );(* Put asdu to the TX fifo *)
		IF fbBuffer.bOk THEN(* Success *)
			fbLog.A_LogHint( sPut := CONCAT( '<=', IEC101ASDU_TO_STRING( txAsdu ) ) );(* Log data (for demonstration purpose only) *)
			eState := e101SState_Init;
		ELSE(* Report send buffer overflow warning *)
			fbLog.A_LogWarning( sPut := '::TX buffer overflow (clock synchronisation activation confirmation)!' );
		END_IF
	(*-----------------------------------------------------------------------------------------*)
	e101SState_GeninAct:(* General interrogation command activation *)
		F_iecCopyStreamToBuffer( ADR( nQoi ), SIZEOF( nQoi ), rxAsdu.info.stream );(* Copy QOI value to local variable *)
		eQoi := BYTE_TO_INT( nQoi );(* Qualifier of interrogation as enumerated type *)
		eState := e101SState_GeninCon;
	(*-----------------------------------------------------------------------------------------*)
	e101SState_GeninCon:(* General interrogation command activation confirmation *)
		txAsdu := rxAsdu;(* Create asdu *)
		txAsdu.ident.eCOT := eIEC870_COT_ACT_CON;(* Send activation confirmation *)
		fbBuffer.TxAddObj( putObj := txAsdu, buffer := buffer );(* Put asdu to the TX fifo *)
		IF fbBuffer.bOk THEN(* Success *)
			fbLog.A_LogHint( sPut := CONCAT( '<=', IEC101ASDU_TO_STRING( txAsdu ) ) );(* Log data (for demonstration purpose only) *)
			
			(* Force transmission of general interrogation data (monitoring data points) *)
			st100.bGenin := TRUE;
			st101.bGenin := TRUE;
			st102.bGenin := TRUE;
			st200.bGenin := TRUE;
			st300.bGenin := TRUE;
			st400.bGenin := TRUE;
			st500.bGenin := TRUE;
			st600.bGenin := TRUE;
			st700.bGenin := TRUE;
			eState := e101SState_GeninTerm;
		ELSE(* Report send buffer overflow warning *)
			fbLog.A_LogWarning( sPut := '::TX buffer overflow (general interrogation activation confirmation)!' );
		END_IF
	(*-----------------------------------------------------------------------------------------*)
	e101SState_GeninTerm:(* General interrogation command activation termination *)
		bGeninWait := st100.bGenin OR st101.bGenin OR st102.bGenin  
					OR st200.bGenin OR st300.bGenin OR st400.bGenin 
					OR st500.bGenin OR st600.bGenin OR st700.bGenin;
		IF NOT bGeninWait THEN(* Transmission of general interrogation data completed *)
			txAsdu := rxAsdu;(* Create asdu *)
			txAsdu.ident.eCOT := eIEC870_COT_ACT_TERM;(* Send activation termination *)
			fbBuffer.TxAddObj( putObj := txAsdu, buffer := buffer );(* Put asdu to the TX fifo *)
			IF fbBuffer.bOk THEN(* Success *)
				fbLog.A_LogHint( sPut := CONCAT( '<=', IEC101ASDU_TO_STRING( txAsdu ) ) );(* Log data (for demonstration purpose only) *)
				eState := e101SState_Init;
			ELSE(* Report send buffer overflow warning *)
				fbLog.A_LogWarning( sPut := '::TX buffer overflow (general interrogation activation termination)!' );
			END_IF
		END_IF
	(*-----------------------------------------------------------------------------------------*)
	e101SState_CoroAct:(* Counter interrogation command activation *)
		F_iecCopyStreamToBuffer( ADR( nQcc ), SIZEOF( nQcc ), rxAsdu.info.stream );(* Copy QCC value to local variable *)
		eRqt:= BYTE_TO_INT( nQcc AND 2#111111 );
		eFrz := BYTE_TO_INT( SHR( nQcc, 6 ) );

		IF eFrz = eIEC870_FRZ_READ THEN(* Read only *)
			;
		ELSIF eFrz = eIEC870_FRZ_FREEZE THEN(* Freeze only *)
			stTxProcData.nBcr800 	:= stProcData.nBcr800;
			stTxProcData.nBcr801 	:= stProcData.nBcr801;
			stTxProcData.nBcr802 	:= stProcData.nBcr802;
		ELSIF eFrz = eIEC870_FRZ_FREEZE_AND_RESET THEN(* Freeze and reset *)
			stTxProcData.nBcr800 	:= stProcData.nBcr800;
			stTxProcData.nBcr801 	:= stProcData.nBcr801;
			stTxProcData.nBcr802 	:= stProcData.nBcr802;
			stProcData.nBcr800 		:= 0;
			stProcData.nBcr801 		:= 0;
			stProcData.nBcr802 		:= 0;
		ELSIF eFrz = eIEC870_FRZ_RESET THEN(* Reset only *)
			stProcData.nBcr800 		:= 0;
			stProcData.nBcr801 		:= 0;
			stProcData.nBcr802 		:= 0;
		END_IF
		eState := e101SState_CoroCon;
	(*-----------------------------------------------------------------------------------------*)
	e101SState_CoroCon:(* Counter interrogation command activation confirmation *)
		txAsdu := rxAsdu;(* Create asdu *)
		txAsdu.ident.eCOT := eIEC870_COT_ACT_CON;(* Send activation confirmation *)
		fbBuffer.TxAddObj( putObj := txAsdu, buffer := buffer );(* Put asdu to the TX fifo *)
		IF fbBuffer.bOk THEN(* Success *)
			fbLog.A_LogHint( sPut := CONCAT( '<=', IEC101ASDU_TO_STRING(txAsdu) ) );(* Log data (for demonstration purpose only) *)
			IF ( eFrz = eIEC870_FRZ_READ ) THEN
				st800.bCoro := TRUE;
				st801.bCoro := TRUE;
				st802.bCoro := TRUE;
				eState := e101SState_CoroTerm;
			ELSE
				IF sysPara.eCoroMode = eIEC870_CoroMode_D THEN(* Counter interrogation MODE D: Force spontaneous data transfer *)
					st800.bSpont := TRUE;
					st801.bSpont := TRUE;
					st802.bSpont := TRUE;
				END_IF
				eState := e101SState_Init;
			END_IF
		ELSE(* Report send buffer overflow warning *)
			fbLog.A_LogWarning( sPut := '::TX buffer overflow (counter interrogation activation confirmation)!' );
		END_IF
	(*-----------------------------------------------------------------------------------------*)
	e101SState_CoroTerm:(* Counter interrogation command activation termination *)
		bCoroWait := st800.bCoro OR st801.bCoro OR st802.bCoro;
		IF NOT bCoroWait THEN(* Transmission of counter interrogation data completed *)
			txAsdu := rxAsdu;(* Create asdu *)
			txAsdu.ident.eCOT := eIEC870_COT_ACT_TERM;(* Send activation termination *)
			fbBuffer.TxAddObj( putObj := txAsdu, buffer := buffer );(* Put asdu to the TX fifo *)
			IF fbBuffer.bOk THEN(* Success *)
				fbLog.A_LogHint( sPut := CONCAT( '<=', IEC101ASDU_TO_STRING(txAsdu) ) );(* Log data (for demonstration purpose only) *)
				eState := e101SState_Init;
			ELSE(* Report send buffer overflow warning *)
				fbLog.A_LogWarning( sPut := '::TX buffer overflow (counter interrogation activation termination)!' );
			END_IF
		END_IF		
	(*-----------------------------------------------------------------------------------------*)
	e101SState_DelayAct:(* Delay acquisition command activation *)
		(* TODO:: *)	
		eState := e101SState_DelayCon;
	(*-----------------------------------------------------------------------------------------*)
	e101SState_DelayCon:(* Delay acquisition command confirmation *)
		txAsdu := rxAsdu;(* Create asdu *)
		txAsdu.ident.eCOT := eIEC870_COT_ACT_CON;(* Send activation confirmation *)
		fbBuffer.TxAddObj( putObj := txAsdu, buffer := buffer );(* Put asdu to the TX fifo *)
		IF fbBuffer.bOk THEN(* Success *)
			fbLog.A_LogHint( sPut := CONCAT( '<=', IEC101ASDU_TO_STRING(txAsdu) ) );(* Log data (for demonstration purpose only) *)
			eState := e101SState_Init;
		ELSE(* Report send buffer overflow warning *)
			fbLog.A_LogWarning( sPut := '::TX buffer overflow (delay acquisition activation confirmation)!' );
		END_IF
		
	(*-----------------------------------------------------------------------------------------*)
	e101SState_DelaySpt:(* Delay acquisition spontaneous data *)		
		(* TODO:: *)	
		eState := e101SState_Init;
	(*-----------------------------------------------------------------------------------------*)
	e101SState_ScsCmdAct:(* Simple single command implementation *)
		F_iecCopyStreamToBuffer( ADR( nSco ), SIZEOF( nSco ), rxAsdu.info.stream );(* Copy SCO value to local variable *)
		IF rxAsdu.ident.eType = C_SC_TA_1 THEN
			 F_iecCopyStreamToBufferByOffset( ADR( tT56 ), 7(* SIZEOF( tT56 ) - 1 *), 1, rxAsdu.info.stream );(* Copy time tag to local variable *)
		END_IF
		eScs := nSco AND 2#1;
		eQu := SHR( nSco, 2 ) AND 2#11111;
		bSE := nSco.7;
		eState := SEL( bSE, e101SState_GenCmdCon, e101SState_GenCmdSel );
	(*-----------------------------------------------------------------------------------------*)
	e101SState_DcsCmdAct:(* Simple double command implementation *)
		F_iecCopyStreamToBuffer( ADR( nDco ), SIZEOF( nDco ), rxAsdu.info.stream );(* Copy DCO value to local variable *)
		IF rxAsdu.ident.eType = C_DC_TA_1 THEN
			 F_iecCopyStreamToBufferByOffset( ADR( tT56 ), 7(* SIZEOF( tT56 ) - 1 *), 1, rxAsdu.info.stream );(* Copy time tag to local variable *)
		END_IF
		eDcs := nDco AND 2#11;
		eQu := SHR( nDco, 2 ) AND 2#11111;
		bSE := nDco.7;
		eState := SEL( bSE, e101SState_GenCmdCon, e101SState_GenCmdSel );
	(*-----------------------------------------------------------------------------------------*)
	e101SState_RcsCmdAct:(* Simple regulating step command implementation *)
		F_iecCopyStreamToBuffer( ADR( nRco ), SIZEOF( nRco ), rxAsdu.info.stream );(* Copy RCO value to local variable *)
		IF rxAsdu.ident.eType = C_RC_TA_1 THEN
			 F_iecCopyStreamToBufferByOffset( ADR( tT56 ), 7(* SIZEOF( tT56 ) - 1 *), 1, rxAsdu.info.stream );(* Copy time tag to local variable *)
		END_IF
		eRcs := nRco AND 2#11;
		eQu := SHR( nRco, 2 ) AND 2#11111;
		bSE := nRco.7;
		eState := SEL( bSE, e101SState_GenCmdCon, e101SState_GenCmdSel );
	(*-----------------------------------------------------------------------------------------*)
	e101SState_BsiCmdAct:(* Simple bitstring command implementation *)
		F_iecCopyStreamToBuffer( ADR( nBsi ), SIZEOF( nBsi ), rxAsdu.info.stream );(* Copy BSI value to local variable *)
		IF rxAsdu.ident.eType = C_BO_TA_1 THEN
			 F_iecCopyStreamToBufferByOffset( ADR( tT56 ), 7(* SIZEOF( tT56 ) - 1 *), 4, rxAsdu.info.stream );(* Copy time tag to local variable *)
		END_IF
		bSE := FALSE;
		eState := SEL( bSE, e101SState_GenCmdCon, e101SState_GenCmdSel );
	(*-----------------------------------------------------------------------------------------*)
	e101SState_NvaCmdAct:(* Simple setpoint command (normalized value) implementation *)
		F_iecCopyStreamToBuffer( ADR( nNva ), SIZEOF( nNva ), rxAsdu.info.stream );(* Copy NVA value to local variable *)
		F_iecCopyStreamToBufferByOffset( ADR( nQos ), SIZEOF( nQos ), 2, rxAsdu.info.stream ); (* Copy QOS value to local variable *)
		IF rxAsdu.ident.eType = C_SE_TA_1 THEN
			 F_iecCopyStreamToBufferByOffset( ADR( tT56 ), 7(* SIZEOF( tT56 ) - 1 *), 4, rxAsdu.info.stream );(* Copy time tag to local variable *)
		END_IF
		eQl := nQos AND 2#1111111;
		bSE := nQos.7;
		eState := SEL( bSE, e101SState_GenCmdCon, e101SState_GenCmdSel );
	(*-----------------------------------------------------------------------------------------*)
	e101SState_SvaCmdAct:(* Simple setpoint command (scalled value) implementation *)
		F_iecCopyStreamToBuffer( ADR( nSva ), SIZEOF( nSva ), rxAsdu.info.stream );(* Copy SVA value to local variable *)
		F_iecCopyStreamToBufferByOffset( ADR( nQos ), SIZEOF( nQos ), 2, rxAsdu.info.stream ); (* Copy QOS value to local variable *)
		IF rxAsdu.ident.eType = C_SE_TB_1 THEN
			 F_iecCopyStreamToBufferByOffset( ADR( tT56 ), 7(* SIZEOF( tT56 ) - 1 *), 4, rxAsdu.info.stream );(* Copy time tag to local variable *)
		END_IF
		eQl := nQos AND 2#1111111;
		bSE := nQos.7;
		eState := SEL( bSE, e101SState_GenCmdCon, e101SState_GenCmdSel );
	(*-----------------------------------------------------------------------------------------*)
	e101SState_R32CmdAct:(* Simple setpoint command (short floating point value) implementation *)
		F_iecCopyStreamToBuffer( ADR( fR32 ), SIZEOF( fR32 ), rxAsdu.info.stream );(* Copy R32 value to local variable *)
		F_iecCopyStreamToBufferByOffset( ADR( nQos ), SIZEOF( nQos ), 4, rxAsdu.info.stream ); (* Copy QOS value to local variable *)
		IF rxAsdu.ident.eType = C_SE_TC_1 THEN
			 F_iecCopyStreamToBufferByOffset( ADR( tT56 ), 7(* SIZEOF( tT56 ) - 1 *), 4, rxAsdu.info.stream );(* Copy time tag to local variable *)
		END_IF
		eQl := nQos AND 2#1111111;
		bSE := nQos.7;
		eState := SEL( bSE, e101SState_GenCmdCon, e101SState_GenCmdSel );
	(*-----------------------------------------------------------------------------------------*)
	e101SState_GenCmdSel:(* Simple implementation of command selection *)
		CASE rxAsdu.ident.eType OF
			C_SC_NA_1, C_SC_TA_1:(* Single command *)
				IF rxAsdu.info.objAddr = 10 THEN
					stProcData.eScs10 		:= eScs;
					stProcData.eQu10 		:= eQu; 
					stProcData.eCtrl10 		:= eIEC870_CMD_SELECT;
				END_IF
			C_DC_NA_1, C_DC_TA_1:(* Double command *)
				IF rxAsdu.info.objAddr = 20 THEN
					stProcData.eDcs20 		:= eDcs;
					stProcData.eQu20 		:= eQu; 
					stProcData.eCtrl20 		:= eIEC870_CMD_SELECT;
				END_IF
			C_RC_NA_1, C_RC_TA_1:(* Regulating step command *)
				IF rxAsdu.info.objAddr = 30 THEN
					stProcData.eRcs30 		:= eRcs;
					stProcData.eQu30 		:= eQu; 
					stProcData.eCtrl30 		:= eIEC870_CMD_SELECT;
				END_IF
			C_SE_NA_1, C_SE_TA_1:(* Set-point command, normalized value *)
				IF rxAsdu.info.objAddr = 50 THEN
					stProcData.nNva50 		:= nNva;
					stProcData.eQl50 		:= eQl; 
					stProcData.eCtrl50 		:= eIEC870_CMD_SELECT;
				END_IF	
			C_SE_NB_1, C_SE_TB_1:(* Set-point command, scalled value *)
				IF rxAsdu.info.objAddr = 60 THEN
					stProcData.nSva60 		:= nSva;
					stProcData.eQl60 		:= eQl; 
					stProcData.eCtrl60 		:= eIEC870_CMD_SELECT;
				END_IF
			C_SE_NC_1, C_SE_TC_1:(* Set-point command, short floating point number *)
				IF rxAsdu.info.objAddr = 70 THEN
					stProcData.fSingle70 	:= fR32;
					stProcData.eQl70 		:= eQl; 
					stProcData.eCtrl70 		:= eIEC870_CMD_SELECT;
				END_IF
		ELSE
			fbLog.A_LogError( sPut := '::Unknown asdu type (command selection)!' );
		END_CASE		
		eState := e101SState_GenCmdCon;	
	(*-----------------------------------------------------------------------------------------*)
	e101SState_GenCmdCon:(* Send command activation confirmation *)
		txAsdu := rxAsdu;(* Create asdu *)
		txAsdu.ident.eCOT := eIEC870_COT_ACT_CON;(* Send activation confirmation *)
		fbBuffer.TxAddObj( putObj := txAsdu, buffer := buffer );(* Put asdu to the TX fifo *)
		IF fbBuffer.bOk THEN(* Success *)
			fbLog.A_LogHint( sPut := CONCAT( '<=', IEC101ASDU_TO_STRING( txAsdu ) ) );(* Log data (for demonstration purpose only) *)
			IF bSE THEN(* => Select *)
				eState := e101SState_Init;
			ELSE(* => Execute *)
				eState := e101SState_GenCmdExe;
			END_IF			
		ELSE(* Report send buffer overflow warning *)
			fbLog.A_LogWarning( sPut := '::TX buffer overflow (command activation confirmation)!' );
		END_IF
	(*-----------------------------------------------------------------------------------------*)
	e101SState_GenCmdExe:(* Simple implementation of command execution *)
		
		CASE rxAsdu.ident.eType OF
			C_SC_NA_1, C_SC_TA_1:(* Single command *)
				IF rxAsdu.info.objAddr = 10 THEN
					stProcData.eScs10 		:= eScs;
					stProcData.eQu10 		:= eQu; 
					stProcData.eCtrl10		:= eIEC870_CMD_EXECUTE;
				END_IF
			C_DC_NA_1, C_DC_TA_1:(* Double command *)
				IF rxAsdu.info.objAddr = 20 THEN
					stProcData.eDcs20 		:= eDcs;
					stProcData.eQu20 		:= eQu; 
					stProcData.eCtrl20 		:= eIEC870_CMD_EXECUTE;
				END_IF
			C_RC_NA_1, C_RC_TA_1:(* Regulating step command *)
				IF rxAsdu.info.objAddr = 30 THEN
					stProcData.eRcs30 		:= eRcs;
					stProcData.eQu30 		:= eQu; 
					stProcData.eCtrl30 		:= eIEC870_CMD_EXECUTE;
					IF eRcs = eIEC870_RCS_DECREMENT THEN
						F_iecDecVTI( stProcData.nVti30 );(* Increment regulating step value *)
					ELSIF eRcs = eIEC870_RCS_INCREMENT THEN
						F_iecIncVTI( stProcData.nVti30 );(* Decrement regulating step value *)
					END_IF
				END_IF
			C_BO_NA_1, C_BO_TA_1:(* Bitstring command *)
				IF rxAsdu.info.objAddr = 40 THEN
					stProcData.nBsi40 		:= nBsi;
					stProcData.eCtrl40 		:= eIEC870_CMD_EXECUTE;
				END_IF
			C_SE_NA_1, C_SE_TA_1:(* Set-point command, normalized value *)
				IF rxAsdu.info.objAddr = 50 THEN
					stProcData.nNva50 		:= nNva;
					stProcData.eQl50 		:= eQl; 
					stProcData.eCtrl50 		:= eIEC870_CMD_EXECUTE;
				END_IF	
			C_SE_NB_1, C_SE_TB_1:(* Set-point command, scalled value *)
				IF rxAsdu.info.objAddr = 60 THEN
					stProcData.nSva60 		:= nSva;
					stProcData.eQl60 		:= eQl; 
					stProcData.eCtrl60 		:= eIEC870_CMD_EXECUTE;
				END_IF
			C_SE_NC_1, C_SE_TC_1:(* Set-point command, short floating point number *)
				IF rxAsdu.info.objAddr = 70 THEN
					stProcData.fSingle70 	:= fR32;
					stProcData.eQl70 		:= eQl; 
					stProcData.eCtrl70 		:= eIEC870_CMD_EXECUTE;
				END_IF
		ELSE				
			fbLog.A_LogError( sPut := '::Unknown asdu type (command execution)!' );
		END_CASE		
		
		IF ( rxAsdu.ident.eType = C_BO_NA_1 ) 
		OR ( rxAsdu.ident.eType = C_BO_TA_1 ) 
		THEN(* Don't send command activation termination for bitstring commands *)
			eState := e101SState_Init;
		ELSE
			eState := e101SState_GenCmdTerm;
		END_IF
	(*-----------------------------------------------------------------------------------------*)
	e101SState_GenCmdTerm:(* Send command activation termination *)
		txAsdu := rxAsdu;(* Create asdu *)
		txAsdu.ident.eCOT := eIEC870_COT_ACT_TERM;(* Send activation termination *)
		fbBuffer.TxAddObj( putObj := txAsdu, buffer := buffer );(* Put asdu to the TX fifo *)
		IF fbBuffer.bOk THEN(* Success *)
			fbLog.A_LogHint( sPut := CONCAT( '<=', IEC101ASDU_TO_STRING( txAsdu ) ) );(* Log data (for demonstration purpose only) *)
			eState := e101SState_Init;
		ELSE(* Report send buffer overflow warning *)
			fbLog.A_LogWarning( sPut := '::TX buffer overflow (command activation termination)!' );
		END_IF
ELSE
	fbLog.A_LogError( sPut := '::Fatal error!' );
	bReset := TRUE;
END_CASE

END_FUNCTION_BLOCK
